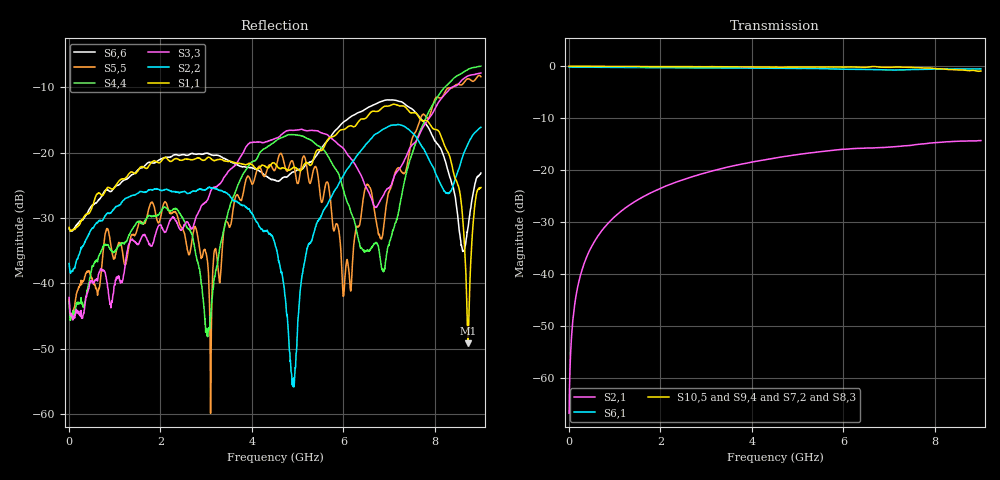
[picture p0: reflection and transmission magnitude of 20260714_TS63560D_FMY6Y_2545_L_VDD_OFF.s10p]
# GHz S DB R 50
! CMT, SN0916, 25263762, 26.7.0
! Date: 15.07.2026 15:21:06
! Data: Format
! Freq S1.1:dB/Ang S1.2:dB/Ang S1.3:dB/Ang S1.4:dB/Ang S1.5:dB/Ang S1.6:dB/Ang S1.7:dB/Ang S1.8:dB/Ang S1.9:dB/Ang S1.10:dB/Ang
!  S2.1:dB/Ang S2.2:dB/Ang S2.3:dB/Ang S2.4:dB/Ang S2.5:dB/Ang S2.6:dB/Ang S2.7:dB/Ang S2.8:dB/Ang S2.9:dB/Ang S2.10:dB/Ang
!  S3.1:dB/Ang S3.2:dB/Ang S3.3:dB/Ang S3.4:dB/Ang S3.5:dB/Ang S3.6:dB/Ang S3.7:dB/Ang S3.8:dB/Ang S3.9:dB/Ang S3.10:dB/Ang
!  S4.1:dB/Ang S4.2:dB/Ang S4.3:dB/Ang S4.4:dB/Ang S4.5:dB/Ang S4.6:dB/Ang S4.7:dB/Ang S4.8:dB/Ang S4.9:dB/Ang S4.10:dB/Ang
!  S5.1:dB/Ang S5.2:dB/Ang S5.3:dB/Ang S5.4:dB/Ang S5.5:dB/Ang S5.6:dB/Ang S5.7:dB/Ang S5.8:dB/Ang S5.9:dB/Ang S5.10:dB/Ang
!  S6.1:dB/Ang S6.2:dB/Ang S6.3:dB/Ang S6.4:dB/Ang S6.5:dB/Ang S6.6:dB/Ang S6.7:dB/Ang S6.8:dB/Ang S6.9:dB/Ang S6.10:dB/Ang
!  S7.1:dB/Ang S7.2:dB/Ang S7.3:dB/Ang S7.4:dB/Ang S7.5:dB/Ang S7.6:dB/Ang S7.7:dB/Ang S7.8:dB/Ang S7.9:dB/Ang S7.10:dB/Ang
!  S8.1:dB/Ang S8.2:dB/Ang S8.3:dB/Ang S8.4:dB/Ang S8.5:dB/Ang S8.6:dB/Ang S8.7:dB/Ang S8.8:dB/Ang S8.9:dB/Ang S8.10:dB/Ang
!  S9.1:dB/Ang S9.2:dB/Ang S9.3:dB/Ang S9.4:dB/Ang S9.5:dB/Ang S9.6:dB/Ang S9.7:dB/Ang S9.8:dB/Ang S9.9:dB/Ang S9.10:dB/Ang
!  S10.1:dB/Ang S10.2:dB/Ang S10.3:dB/Ang S10.4:dB/Ang S10.5:dB/Ang S10.6:dB/Ang S10.7:dB/Ang S10.8:dB/Ang S10.9:dB/Ang S10.10:dB/Ang
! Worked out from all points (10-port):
!   2001 points, 10 MHz to 9 GHz, reference 50 ohm
!   strongest paths, dB at 10 MHz, 2.257 GHz, 4.505 GHz, 6.753 GHz, 9 GHz:
!     S10,5: -0.1, -0.2, -0.2, -0.2, -1.0
!     S9,4: -0.1, -0.2, -0.4, -0.4, -1.5
!     S7,2: -0.1, -0.3, -0.4, -0.6, -0.6
!     S8,3: -0.1, -0.2, -0.4, -0.4, -1.3
!     S6,1: -0.2, -0.4, -0.5, -0.7, -0.6
!     S2,1: -66.8, -22.7, -17.7, -15.7, -14.4
!   lowest |S11| = -49.2 dB at 8.721 GHz (marker M1), VSWR 1.01, Z = 49.9 + j0.325 ohm
!   |S11| at or under -10 dB: start of sweep to end of sweep
